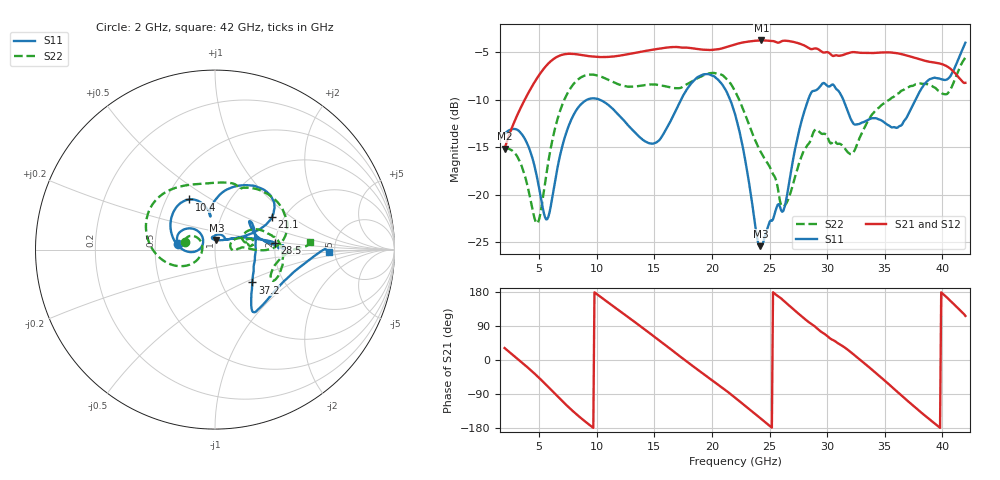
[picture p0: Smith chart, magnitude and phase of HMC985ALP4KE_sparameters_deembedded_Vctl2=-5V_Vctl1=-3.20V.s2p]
!s2p File: Measurements: S11, S21, S12, S22
# GHz S dB R 50.0
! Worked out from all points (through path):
!   401 points, 2 GHz to 42 GHz, reference 50 ohm
!   highest |S21| = -3.74 dB at 24.3 GHz (marker M1); lowest = -15.1 dB at 2 GHz (marker M2)
!   lowest |S11| = -25.4 dB at 24.2 GHz (marker M3), VSWR 1.11, Z = 50.5 + j5.39 ohm
!   |S11| at or under -10 dB: start of sweep to 9.125 GHz; 10.3 GHz to 17.31 GHz (7.016 GHz wide, 50.8 % of centre); 21.58 GHz to 28.35 GHz (6.766 GHz wide, 27.1 % of centre)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
!   |S22| runs from -23.0 to -5.5 dB; largest |S21 - S12| = 0.00086
!   S11 on the Smith chart (normalised r, x): 2 GHz: 0.65, +0.04; 10.4 GHz: 0.65, +0.40; 21.1 GHz: 1.74, +0.72; 28.5 GHz: 1.99, +0.17; 37.2 GHz: 1.40, -0.55; 42 GHz: 4.44, -0.19
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2  -13.55 171.4  -15.13 31.5  -15.14 31.5  -15.12 165.5
3.6  -13.79 146.4  -10.33 -9.1  -10.33 -9.1  -17.38 147.0
4.9  -18.66 132.3  -7.55 -44.5  -7.56 -44.5  -22.90 -177.4
5.8  -22.30 168.8  -6.16 -71.4  -6.16 -71.4  -16.45 -148.6
7.1  -14.45 177.9  -5.21 -111.2  -5.22 -111.2  -10.22 -171.0
8.7  -10.37 142.9  -5.27 -155.1  -5.28 -155.1  -7.58 155.6
10.4  -10.05 117.3  -5.49 164.9  -5.49 165.0  -7.56 128.5
13.2  -13.27 99.2  -5.08 102.4  -5.08 102.4  -8.59 91.1
15.4  -14.27 98.7  -4.61 52.2  -4.61 52.2  -8.44 71.7
18  -8.58 71.5  -4.52 -8.3  -4.52 -8.2  -8.23 62.9
21.1  -8.78 29.6  -4.49 -77.7  -4.49 -77.7  -7.60 15.9
22  -11.48 24.4  -4.16 -99.3  -4.16 -99.2  -9.06 4.0
24.2  -25.39 81.6  -3.74 -153.6  -3.74 -153.5  -15.40 3.5
24.3  -25.33 89.1  -3.74 -156.1  -3.74 -156.0  -15.63 4.0
26.2  -21.66 41.8  -3.77 157.2  -3.77 157.3  -21.22 12.0
28.5  -9.52 6.5  -4.61 97.9  -4.61 98.0  -14.43 17.7
28.7  -9.10 3.0  -4.65 94.0  -4.65 94.0  -13.75 17.1
32.4  -12.60 25.1  -4.97 11.9  -4.97 11.9  -15.26 26.4
35.4  -12.72 11.7  -5.00 -65.2  -5.00 -65.1  -9.98 15.4
37.2  -11.13 -41.3  -5.42 -113.5  -5.42 -113.5  -8.56 0.5
39.7  -7.74 -52.4  -6.15 -176.5  -6.15 -176.4  -9.06 -28.0
42  -3.98 -1.2  -8.20 116.3  -8.21 116.4  -5.51 4.4
